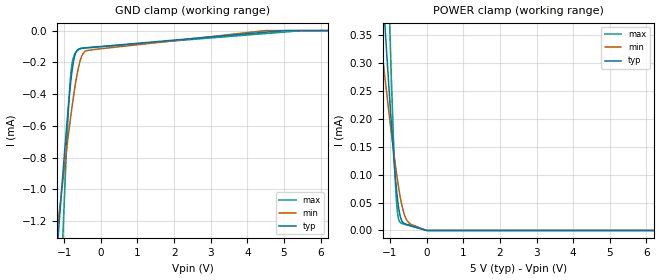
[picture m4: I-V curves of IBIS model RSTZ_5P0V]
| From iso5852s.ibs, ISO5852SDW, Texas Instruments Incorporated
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|   Model RSTZ_5P0V
[Model]   RSTZ_5P0V
Model_type   Input
Vinl = 1.5
Vinh = 3.5
|   typ   min   max
|   (nom PVT)   (slow PVT)   (fast PVT)
C_comp   0.02p   0.01p   0.03p
| Where   nom PVT is  Nominal Process, 5.0V, 27C
|   Fast PVT is Strong Process, 5.5V, -40C
|   Slow PVT is Weak Process, 4.5V, 150C
[Model spec]
|subparameter
Vinl   1.50   1.35   1.65
Vinh   3.50   3.15   3.85
[Voltage Range]   5.0   4.5   5.5
[Temperature Range]   27   150   -40
[Power Clamp Reference]   5.0   4.5   5.5
[GND Clamp Reference]   0   0   0
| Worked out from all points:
|   GND clamp passes 1 mA (typ) near -1.07 V on its own axis
[GND Clamp]
|   Voltage   I(typ)   I(min)   I(max)
-5V       -14.18mA   -9.454mA   -28.61mA
-1.235V   -1.517mA   -1.344mA   -2.531mA
-1.13V    -1.187mA   -1.131mA   -1.86mA
-1.04V    -911.7uA   -951.7uA   -1.312mA
-1.025V   -866.8uA   -922.2uA   -1.224mA
-890mV    -485.5uA   -663.8uA   -515.1uA
-815mV    -308.3uA   -528.5uA   -261uA
-710mV    -155.1uA   -358.1uA   -147.4uA
-575mV    -113.7uA   -197.2uA   -115.4uA
-395mV    -108uA     -126.7uA   -109.1uA
4.495V    -10.1uA    -114.8nA   -18.6uA
10V       0A         0A         0A
[POWER Clamp]
|   Voltage   I(typ)   I(min)   I(max)
-5V       185.6mA    66.98mA    302.3mA
-3.35V    2.813mA    1.63mA     6.063mA
-1.25V    483.8uA    338.2uA    914.2uA
-1.13V    357.7uA    268.3uA    636.2uA
-1.01V    236.1uA    200.4uA    369.5uA
-890mV    124.5uA    136uA      136.4uA
-830mV    77.83uA    106.1uA    58.01uA
-770mV    43.14uA    78.95uA    21.39uA
-680mV    17.24uA    46.15uA    12.7uA
-470mV    9.396uA    12.8uA     8.691uA
-5mV      90.25nA    115.3nA    84.74nA
10V       0A         0A         0A
